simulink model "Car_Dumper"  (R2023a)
settings: Solver=VariableStepAuto  StartTime=0.0  StopTime=10.0  RelTol=1e-3
libraries: fl_lib x10, nesl_utility x2

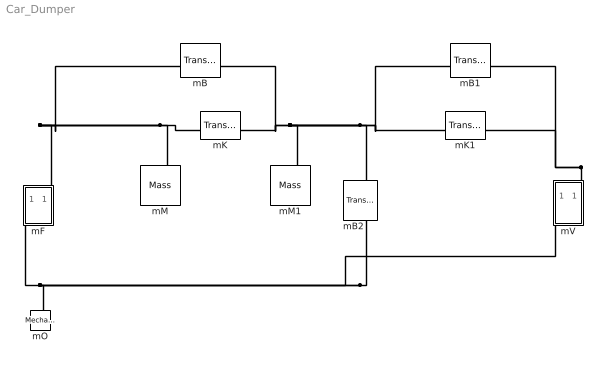
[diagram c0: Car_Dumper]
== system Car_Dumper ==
  mB : fl_lib/Mechanical/Translational Elements/Translational Damper  D=100 N*s/m  v_specify=off  v_priority=None  v=0 m/s  v_nominal_specify=off  v_nominal_unit=m/s  v_nominal_value=1  f_specify=off  f_priority=None  f=0 N  f_nominal_specify=off  f_nominal_unit=N  f_nominal_value=1
  mB1 : fl_lib/Mechanical/Translational Elements/Translational Damper  D=100 N*s/m  v_specify=off  v_priority=None  v=0 m/s  v_nominal_specify=off  v_nominal_unit=m/s  v_nominal_value=1  f_specify=off  f_priority=None  f=0 N  f_nominal_specify=off  f_nominal_unit=N  f_nominal_value=1
  mB2 : fl_lib/Mechanical/Translational Elements/Translational Damper  D=100 N*s/m  v_specify=off  v_priority=None  v=0 m/s  v_nominal_specify=off  v_nominal_unit=m/s  v_nominal_value=1  f_specify=off  f_priority=None  f=0 N  f_nominal_specify=off  f_nominal_unit=N  f_nominal_value=1
  mF : Subsystem  mask{mF='Fa'}
      mask prompts: mF "Output variable"
  mK : fl_lib/Mechanical/Translational Elements/Translational Spring  spr_rate=1000 N/m  v_specify=off  v_priority=None  v=0 m/s  v_nominal_specify=off  v_nominal_unit=m/s  v_nominal_value=1  f_specify=off  f_priority=None  f=0 N  f_nominal_specify=off  f_nominal_unit=N  f_nominal_value=1  x_specify=off  x_priority=High  x=0 m  x_nominal_specify=off  x_nominal_unit=m  x_nominal_value=1
  mK1 : fl_lib/Mechanical/Translational Elements/Translational Spring  spr_rate=1000 N/m  v_specify=off  v_priority=None  v=0 m/s  v_nominal_specify=off  v_nominal_unit=m/s  v_nominal_value=1  f_specify=off  f_priority=None  f=0 N  f_nominal_specify=off  f_nominal_unit=N  f_nominal_value=1  x_specify=off  x_priority=High  x=0 m  x_nominal_specify=off  x_nominal_unit=m  x_nominal_value=1
  mM : fl_lib/Mechanical/Translational Elements/Mass  mass=1 kg  num_ports=foundation.enum.numPorts2.one  v_specify=off  v_priority=High  v=0 m/s  v_nominal_specify=off  v_nominal_unit=m/s  v_nominal_value=1  f_specify=off  f_priority=None  f=0 N  f_nominal_specify=off  f_nominal_unit=N  f_nominal_value=1
  mM1 : fl_lib/Mechanical/Translational Elements/Mass  mass=1 kg  num_ports=foundation.enum.numPorts2.one  v_specify=off  v_priority=High  v=0 m/s  v_nominal_specify=off  v_nominal_unit=m/s  v_nominal_value=1  f_specify=off  f_priority=None  f=0 N  f_nominal_specify=off  f_nominal_unit=N  f_nominal_value=1
  mO : fl_lib/Mechanical/Translational Elements/Mechanical Translational Reference
  mV : Subsystem  mask{mV='Va'}
      mask prompts: mV "Output variable"
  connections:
  mB2/RConn1 -- mV/RConn1 -- mF/RConn1 -- mO/LConn1
  mK/LConn1 -- mM/LConn1 -- mB/LConn1 -- mF/LConn1
  mB2/LConn1 -- mB1/LConn1 -- mK1/LConn1 -- mB/RConn1 -- mK/RConn1 -- mM1/LConn1
  mV/LConn1 -- mB1/RConn1 -- mK1/RConn1

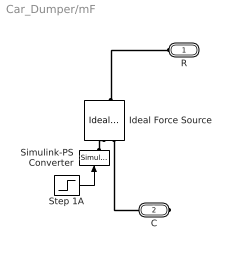
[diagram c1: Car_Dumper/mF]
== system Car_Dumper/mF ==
  Ideal Force Source : fl_lib/Mechanical/Mechanical Sources/Ideal Force Source
  Simulink-PS Converter : nesl_utility/Simulink-PS Converter  PhysicalDomain=network_engine_domain  SubClassName=ps_input  LeftPortType=input  RightPortType=output  PseudoPeriodic=off  Frequencies=[]  NoiseDistribution=none  NoiseParameters=[]  Unit=1  AffineConversion=off  FilteringAndDerivatives=zero  SimscapeFilterOrder=1  InputFilterTimeConstant=.001  UdotUserProvided=0
  Step 1A : Step  After=100  SampleTime=0
  R : PMIOPort  Side=Left
  C : PMIOPort  Port=2  Side=Right
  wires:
  Step 1A/1 -> Simulink-PS Converter/1
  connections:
  Simulink-PS Converter/RConn1 -- Ideal Force Source/RConn1
  Ideal Force Source/LConn1 -- R/RConn1
  Ideal Force Source/RConn2 -- C/RConn1

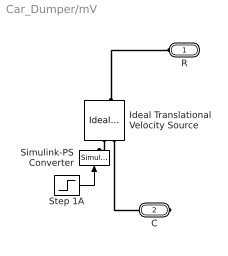
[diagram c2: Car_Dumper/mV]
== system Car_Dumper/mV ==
  Ideal Translational Velocity Source : fl_lib/Mechanical/Mechanical Sources/Ideal Translational Velocity Source
  Simulink-PS Converter : nesl_utility/Simulink-PS Converter  PhysicalDomain=network_engine_domain  SubClassName=ps_input  LeftPortType=input  RightPortType=output  PseudoPeriodic=off  Frequencies=[]  NoiseDistribution=none  NoiseParameters=[]  Unit=1  AffineConversion=off  FilteringAndDerivatives=zero  SimscapeFilterOrder=1  InputFilterTimeConstant=.001  UdotUserProvided=0
  Step 1A : Step  After=100  SampleTime=0
  R : PMIOPort  Side=Left
  C : PMIOPort  Port=2  Side=Right
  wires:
  Step 1A/1 -> Simulink-PS Converter/1
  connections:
  Ideal Translational Velocity Source/RConn1 -- Simulink-PS Converter/RConn1
  Ideal Translational Velocity Source/LConn1 -- R/RConn1
  Ideal Translational Velocity Source/RConn2 -- C/RConn1
